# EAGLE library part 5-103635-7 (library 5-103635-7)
Body Features: Primary Product Color Black | Configuration Features: Number of Rows 1 | Number of Positions 8 | PCB Mount Orientation Right Angle | Contact Features: PCB Contact Termination Area Plating Material Thickness 2.54 MICM | Contact Type Pin | Mating Square Post Dimension .64 MM | Contact Mating Area Plating Material Thickness .381 MICM | Contact Shape & Form Square | Mating Square Post Dimension .025 INCH | PCB Contact Termination Area Plating Material Finish Matte | Contact Mating Area Plating Ma Source: Datasheet
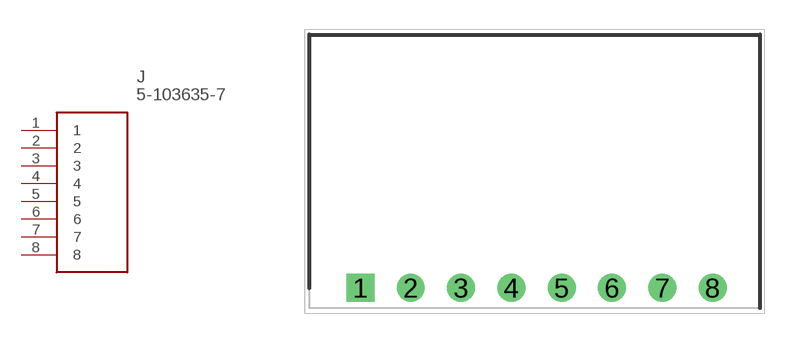
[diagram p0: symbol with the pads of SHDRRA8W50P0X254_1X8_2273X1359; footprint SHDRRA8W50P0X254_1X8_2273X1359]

Designator prefix J

## 5-103635-7 (Description: Body Features: Primary Product Color Black | Configuration Features: Number of Rows 1 | Number of Positions 8 | PCB Mount Orientation Right Angle | Contact Features: PCB Contact Termination Area Plating Material Thickness 2.54 MICM | Contact Type Pin | Mating Square Post Dimension .64 MM | Contact Mating Area Plating Material Thickness .381 MICM | Contact Shape & Form Square | Mating Square Post Dimension .025 INCH | PCB Contact Termination Area Plating Material Finish Matte | Contact Mating Area Plating Ma; Height: 7.41mm; Manufacturer_Name: TE Connectivity; Manufacturer_Part_Number: 5-103635-7; Mouser_Part_Number: 571-5-103635-7; Mouser_Price-Stock: https://www.mouser.co.uk/ProductDetail/TE-Connectivity-AMP/5-103635-7?qs=zx8qD9ablb2pkVx90XSXJA%3D%3D)  [SHDRRA8W50P0X254_1X8_2273X1359]
1  1
2  2
3  3
4  4
5  5
6  6
7  7
8  8

## Footprint SHDRRA8W50P0X254_1X8_2273X1359 (pad centres in mm)
5-103635-7
drill 0.9 pad 1.35 square: 1 0,0
drill 0.9 pad 1.35: 2 2.54,0; 3 5.08,0; 4 7.62,0; 5 10.16,0; 6 12.7,0; 7 15.24,0; 8 17.78,0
